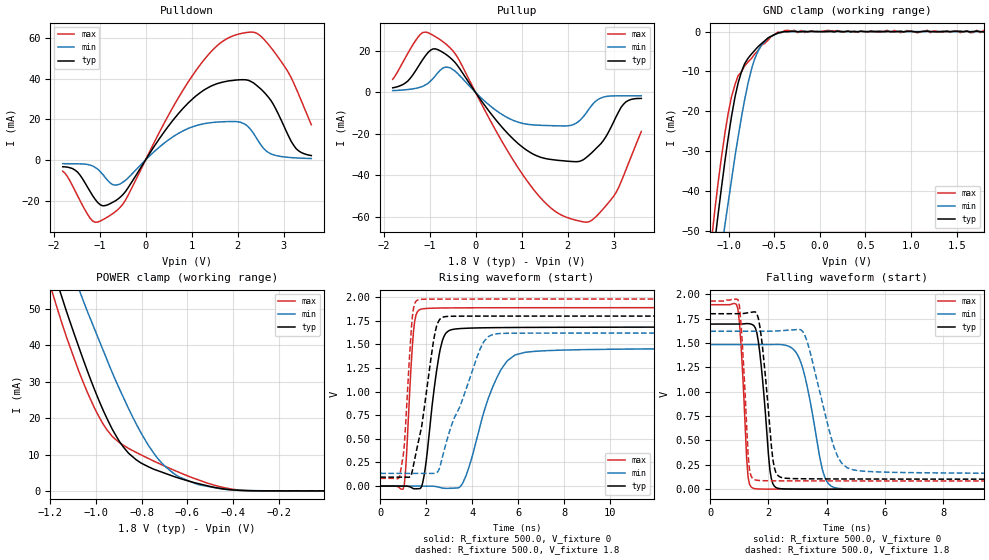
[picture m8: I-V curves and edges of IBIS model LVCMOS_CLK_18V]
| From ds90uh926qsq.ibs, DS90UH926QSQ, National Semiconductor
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[Model] LVCMOS_CLK_18V
Model_type 3-state
Enable Active-High
Vmeas = 0.9V
Cref = 0.0pF
Rref = 1.0e10
Vref = 0.0V
C_comp   2.75pF   2.32pF   3.18pF
[Voltage Range]   1.8V   1.62V   1.98V
[Temperature Range]   25.0   130.0   -40.0
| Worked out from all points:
|   slope of the pulldown table from 0 to 0.27 V, typ, clamps not added: 28.5 ohm
|   slope of the pullup table from 0 to 0.27 V, typ, clamps not added: 32.2 ohm
|   GND clamp passes 1 mA (typ) near -0.52 V on its own axis
|   POWER clamp passes 1 mA (typ) near -0.48 V on its own axis
|   rising waveform, R_fixture 500.0, V_fixture 0: 20-80 % time 500ps typ, 1.15ns min, 253ps max; typ from 0 V to 1.69 V
|   falling waveform, R_fixture 500.0, V_fixture 0: 20-80 % time 286ps typ, 558ps min, 191ps max; typ from 1.69 V to 0 V
|   rising waveform, R_fixture 500.0, V_fixture 1.8: 20-80 % time 640ps typ, 1.31ns min, 278ps max; typ from 0.094 V to 1.8 V
|   falling waveform, R_fixture 500.0, V_fixture 1.8: 20-80 % time 307ps typ, 740ps min, 196ps max; typ from 1.8 V to 0.1 V
[GND Clamp]
-1.8V     -189.3mA   -183.9mA   -199.6mA
-1.186V   -59.78mA   -73.23mA   -52.22mA
-1.148V   -52.22mA   -66.57mA   -44.27mA
-1.115V   -45.93mA   -61.06mA   -38.02mA
-1.038V   -32.25mA   -48.23mA   -25.28mA
-966.7mV  -21.2mA    -37.12mA   -16.3mA
-857.1mV  -9.999mA   -21.31mA   -10.06mA
-785.8mV  -6.684mA   -12.93mA   -7.621mA
-714.5mV  -4.758mA   -6.909mA   -5.649mA
-566.5mV  -1.581mA   -1.669mA   -2.157mA
-347.2mV  -17.27uA   -50.86uA   302.6uA
1.796V    -108.1uA   0A         267.9uA
[POWER Clamp]
-1.8V     189.4mA    185.2mA    199.2mA
-1.186V   60.43mA    74.18mA    53.54mA
-1.148V   52.96mA    67.56mA    45.82mA
-1.06V    36.85mA    53.03mA    30.51mA
-966.7mV  21.93mA    38.4mA     18.2mA
-879mV    12mA       25.6mA     12.52mA
-769.3mV  6.604mA    12.45mA    8.883mA
-714.5mV  5.229mA    7.863mA    7.266mA
-659.7mV  3.981mA    4.813mA    5.734mA
-550.1mV  1.973mA    1.699mA    3mA
-402mV    276.4uA    274.3uA    458.6uA
-1.827mV  668.5nA    4.878uA    -4.278uA
[Pullup]
-1.8V     2.23mA     888.9uA    6.331mA
-1.148V   15.9mA     2.949mA    28.97mA
-714.5mV  19.39mA    11.73mA    24.62mA
-385.6mV  12.79mA    9.084mA    16.76mA
376.4mV   -11.46mA   -7.548mA   -15.88mA
1.034V    -26.7mA    -15.04mA   -40.06mA
1.687V    -32.54mA   -16.08mA   -56.75mA
2.29V     -33.06mA   -12.97mA   -62.32mA
2.613V    -27.17mA   -4.13mA    -60.07mA
2.997V    -14.32mA   -1.661mA   -50.22mA
3.271V    -4.454mA   -1.635mA   -37.09mA
3.6V      -2.89mA    -1.622mA   -18.83mA
[Pulldown]
-1.8V     -3.361mA   -1.851mA   -5.551mA
-1.477V   -6.017mA   -1.938mA   -17.69mA
-1.148V   -17.69mA   -2.991mA   -30.14mA
-928.3mV  -22.62mA   -7.158mA   -29.44mA
-659.7mV  -20.21mA   -12.45mA   -25.56mA
924.7mV   28.02mA    15.47mA    38.35mA
1.577V    37.73mA    18.67mA    56.7mA
2.125V    39.51mA    17.97mA    62.5mA
2.454V    35.89mA    9.053mA    61.81mA
2.778V    27.24mA    2.523mA    53.73mA
3.271V    5.516mA    982.4uA    35.14mA
3.6V      2.128mA    687.2uA    17.3mA
[Rising Waveform]
R_fixture=500.0
V_fixture=0
V_fixture_min=0
V_fixture_max=0
0s        24.04nV    644nV      3.943nV
1ns       17.24uV    666.5nV    -30.77mV
1.1ns     80.87uV    652.8nV    163.5mV
1.45ns    -28.12mV   634.9nV    1.649V
1.85ns    39.97mV    -5.919uV   1.877V
2.6ns     1.44V      -15.52mV   1.885V
3.25ns    1.663V     -21.53mV   1.887V
5.1ns     1.678V     1.162V     1.888V
6.35ns    1.68V      1.418V     1.888V
49.98ns   1.686V     1.466V     1.89V
[Falling Waveform]
R_fixture=500.0
V_fixture=0
V_fixture_min=0
V_fixture_max=0
0s        1.694V     1.483V     1.893V
950ps     1.694V     1.483V     1.848V
1.3ns     1.699V     1.483V     122.1mV
1.55ns    1.654V     1.483V     4.45mV
2.05ns    196.6mV    1.483V     398.6uV
2.4ns     5.276mV    1.484V     235.2uV
3.1ns     547.7uV    1.311V     127.6uV
3.85ns    268.6uV    204.4mV    84.3uV
4.4ns     191.1uV    8.446mV    67.39uV
49.98ns   6.648uV    17.46uV    2.333uV
[Rising Waveform]
R_fixture=500.0
V_fixture=1.8
V_fixture_min=1.62
V_fixture_max=1.98
0s        94.39mV    134.3mV    81.5mV
850ps     94.39mV    134.3mV    111.8mV
1.05ns    94.43mV    134.3mV    442.2mV
1.4ns     167.2mV    134.3mV    1.802V
1.7ns     511.4mV    134.3mV    1.975V
2.3ns     1.51V      133.7mV    1.979V
2.55ns    1.751V     170.6mV    1.98V
4.35ns    1.8V       1.454V     1.98V
5.1ns     1.8V       1.613V     1.98V
49.98ns   1.8V       1.62V      1.98V
[Falling Waveform]
R_fixture=500.0
V_fixture=1.8
V_fixture_min=1.62
V_fixture_max=1.98
0s        1.8V       1.62V      1.93V
950ps     1.8V       1.62V      1.944V
1.35ns    1.813V     1.62V      195.3mV
1.65ns    1.755V     1.62V      89.6mV
2.15ns    308.1mV    1.62V      85.61mV
2.55ns    113.7mV    1.628V     85.17mV
3.2ns     106.6mV    1.607V     84.83mV
4.35ns    104.6mV    354.3mV    84.53mV
5.1ns     104mV      189mV      84.42mV
49.98ns   100.3mV    151mV      83.51mV
[Ramp]
R_load = 500.0
dV/dt_r   1.011718E0/5E-10   8.7965E-1/1.15E-9   1.133986E0/2.5E-10
dV/dt_f   1.019847E0/3.5E-10   8.813788E-1/7.5E-10   1.137891E0/2E-10
